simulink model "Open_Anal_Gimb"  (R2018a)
settings: Solver=ode5  StartTime=0.0  StopTime=25000  FixedStep=Ts  RelTol=1e-3  EnableMultiTasking=on
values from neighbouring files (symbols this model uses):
  Kq1 = I22*ww^2 - 3*wo2*(I11-I33)    [start.m]    (also in run.m)
  Kq2 = 2*I22*zet*ww    [start.m]    (also in run.m)
  Kqi = 0.0005    [start.m]    (also in run.m)
  Kr1 = (0.1*I11*I33*zet^2/Hy0) - sqrt( ((0.01^zet^4*I11^2*I33^2)/Hy0^2)+(4*I11*I33*zet^2) )    [start.m]    (also in run.m)
  Kr2 = 0.05*Kr1    [start.m]    (also in run.m)
  Kr3 = 0.04*zet*(Kr2-Hy0) * sqrt(abs(Hy0/(I11*I33)))    [start.m]    (also in run.m)
  Ts = 0.01    [start.m]    (also in run.m = 0.001; runf.m = 0.0005)
undefined symbols (not defined in the file or in its folder): Avf, Bvf, Cvf, den, DiscIntNeverNeededParam, Dvf, num, RW_Steering
libraries: simulink x3

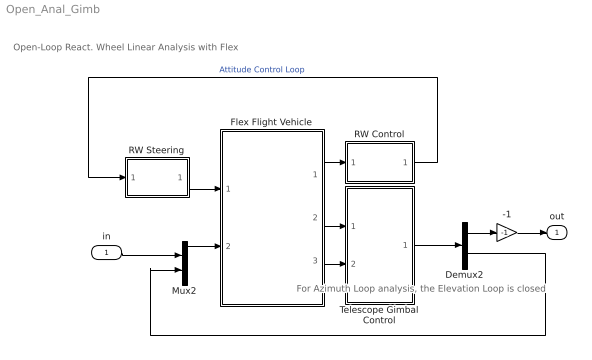
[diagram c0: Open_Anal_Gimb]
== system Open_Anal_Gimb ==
  note: For Azimuth Loop analysis, the Elevation Loop is closed
  note: Open-Loop React. Wheel Linear Analysis with Flex
  in : Inport
  -1 : Gain  Gain=-1
  Demux2 : Demux  Outputs=2
  Flex Flight Vehicle : Subsystem
  Mux2 : Mux  Inputs=2
  RW Control : Subsystem
  RW Steering : Subsystem
  Telescope Gimbal Control : Subsystem
  out : Outport
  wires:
  -1/1 -> out/1
  Flex Flight Vehicle/1(atti) -> RW Control/1(atti)
  RW Steering/1(Twi) -> Flex Flight Vehicle/1(Trw(i))
  Mux2/1 -> Flex Flight Vehicle/2(Tgimb)
  RW Control/1(Tc) -> RW Steering/1(Trwc)  "Attitude Control Loop"
  Flex Flight Vehicle/2(alfa) -> Telescope Gimbal Control/1(Gimb)
  Flex Flight Vehicle/3(alfad) -> Telescope Gimbal Control/2(Grate)
  Telescope Gimbal Control/1(GTrq) -> Demux2/1
  in/1 -> Mux2/1
  Demux2/1 -> -1/1
  Demux2/2 -> Mux2/2

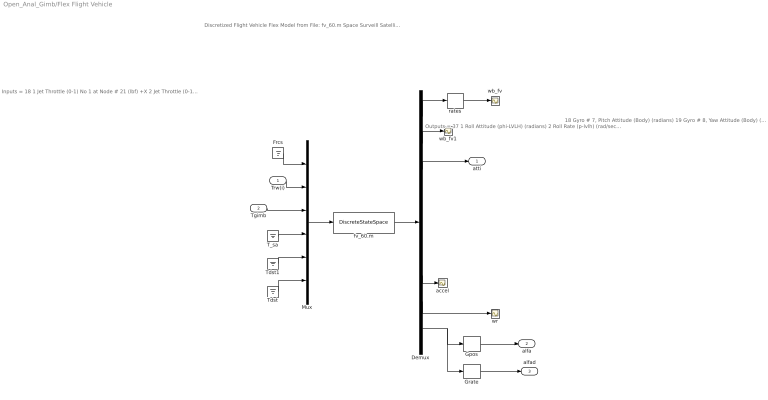
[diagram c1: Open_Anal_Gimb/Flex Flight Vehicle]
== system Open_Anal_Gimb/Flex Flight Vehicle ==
  note: Discretized Flight Vehicle Flex Model from File: fv_60.m Space Surveill Satellite with RCS and Reaction Wheels (Gimbals, 60 Modes, Z-Transf)
  note: Inputs = 18 1 Jet Throttle (0-1) No 1 at Node # 21 (lbf) +X 2 Jet Throttle (0-1) No 2 at Node # 22 (lbf) +X 3 Jet Throttle (0-1) No 3 at Node # 23 (lbf) +Y 4 Jet Throttle (0-1) No 4 at Node # 24 (lbf) -Y 5 Jet Throttle (0-1) No 5 at Node # 25 (lbf) -Y 6 Jet Throttle (0-1) No 6 at Node # 26 (lbf) +Y 7 Jet Throttle (0-1) No 7 at Node # 27 (lbf) +X 8 React-Wheel No 1 Torque to Spacecraft (ft-lb) 9 React-Wheel No 2 Torque to Spacecraft (ft-lb) 10 React-Wheel No 3 Torque to Spacecraft (ft-lb) 11 Elevation Trqu at Gimbal No 1 (ft-lb) 12 Azimuth Torque at Gimbal No 2 (ft-lb) 13 Rght SA Torque at Gimbal No 3 (ft-lb) 14 Left SA Torque at Gimbal No 4 (ft-lb) 15 Ext Torque Input 1 (ft-lb), dir: 1.00 0.00 0.00 16 Ext Torque Input 2 (ft-lb), dir: 0.00 1.00 0.00 17 Ext Torque Input 3 (ft-lb), dir: 0.00 0.00 1.00 18 Ext Torque Direct.=( 0.1970 -0.5964 -0.7782)
  note: Outputs = 37 1 Roll Attitude (phi-LVLH) (radians) 2 Roll Rate (p-lvlh) (rad/sec) 3 Pitch Attitude (thet-LVLH) (radians) 4 Pitch Rate (q-lvlh) (rad/sec) 5 Yaw Attitude (psi-LVLH) (radians) 6 Yaw Rate (r-lvlh) (rad/sec) 7 Angle of attack, alfa, (radians) 8 Angle of sideslip, beta, (radian) 9 Change in Altitude, delta-h, (feet) 10 Forward Acceleration (V-dot) (ft/sec) 11 Cross Range Velocity (Vcr) (ft/sec) 12 Rate-Gyro # 1, Roll Rate (Body) (rad/sec) 13 Rate-Gyro # 2, Pitch Rate (Body) (rad/sec) 14 Rate-Gyro # 3, Yaw Rate (Body) (rad/sec) 15 Gyro # 4, Roll Attitude (Body) (radians) 16 Gyro # 5, Pitch Attitude (Body) (radians) 17 Gyro # 6, Yaw Attitude (Body) (radians)
  note: 18 Gyro # 7, Pitch Attitude (Body) (radians) 19 Gyro # 8, Yaw Attitude (Body) (radians) 20 Gyro # 9, Pitch Attitude (Body) (radians) 21 Gyro # 10, Yaw Attitude (Body) (radians) 22 Gyro # 11, Roll Attitude (Body) (radians) 23 Gyro # 12, Pitch Attitude (Body) (radians) 24 Gyro # 13, Yaw Attitude (Body) (radians) 25 Translat. Accelerom # 1, (along X), (ft/sec^2) 26 Translat. Accelerom # 2, (along Y), (ft/sec^2) 27 Reaction Wheel # 1 Rate (rpm) relative to vehicle 28 Reaction Wheel # 2 Rate (rpm) relative to vehicle 29 Reaction Wheel # 3 Rate (rpm) relative to vehicle 30 Rotation Angle at Elevati Gimbal No 1 31 Rotation Rate at Elevati Gimbal No 1 32 Rotation Angle at Azimuth Gimbal No 2 33 Rotation Rate at Azimuth Gimbal No 2 34 Rotation Angle at Rght SA Gimbal No 3 35 Rotation Rate at Rght SA Gimbal No 3 36 Rotation Angle at Left SA Gimbal No 4 37 Rotation Rate at Left SA Gimbal No 4
  Trw(i) : Inport
  Tgimb : Inport  Port=2
  Demux : Demux  Outputs=[11, 3, 3, 2, 2, 3, 2, 3, 8]
  Frcs : Ground
  Gpos : Selector  InputPortWidth=8  IndexOptions=Index vector (dialog)  Indices=[1,3]  OutputSizes=1
  Grate : Selector  InputPortWidth=8  IndexOptions=Index vector (dialog)  Indices=[2,4]  OutputSizes=1
  Mux : Mux  Inputs=[7,3,2,2,3,1]
  T_sa : Ground
  Tdst : Ground
  Tdst1 : Ground
  accel : Scope
  fv_60.m : DiscreteStateSpace  A=Avf  B=Bvf  C=Cvf  D=Dvf  SampleTime=Ts
  rates : Selector  InputPortWidth=11  IndexOptions=Index vector (dialog)  Indices=[2, 4, 6]  OutputSizes=1
  wb_fv : Scope
  wb_fv1 : Scope
  wr : Scope
  atti : Outport
  alfa : Outport  Port=2
  alfad : Outport  Port=3
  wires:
  Mux/1 -> fv_60.m/1
  Frcs/1 -> Mux/1
  Trw(i)/1 -> Mux/2
  Demux/8 -> wr/1
  Demux/1 -> rates/1
  rates/1 -> wb_fv/1
  Demux/9 -> Gpos/1, Grate/1
  Demux/2 -> wb_fv1/1
  Demux/7 -> accel/1
  Demux/3 -> atti/1
  Grate/1 -> alfad/1
  Gpos/1 -> alfa/1
  Tgimb/1 -> Mux/3
  Tdst1/1 -> Mux/5
  T_sa/1 -> Mux/4
  Tdst/1 -> Mux/6
  fv_60.m/1 -> Demux/1

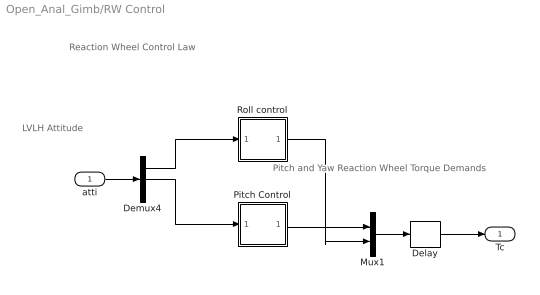
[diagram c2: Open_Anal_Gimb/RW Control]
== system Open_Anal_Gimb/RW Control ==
  note: Reaction Wheel Control Law
  note: LVLH Attitude
  note: Pitch and Yaw Reaction Wheel Torque Demands
  atti : Inport
  Delay : Delay  DelayLength=1  InputProcessing=Inherited  SampleTime=Ts
  Demux4 : Demux  Outputs=3
  Mux1 : Mux  Inputs=2
  Pitch Control : Subsystem
  Roll control : Subsystem
  Tc : Outport
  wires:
  Delay/1 -> Tc/1
  Roll control/1(Tcz) -> Mux1/2
  Mux1/1 -> Delay/1
  atti/1 -> Demux4/1
  Demux4/2 -> Pitch Control/1(the)
  Pitch Control/1(Tcy) -> Mux1/1
  Demux4/1 -> Roll control/1(phi)

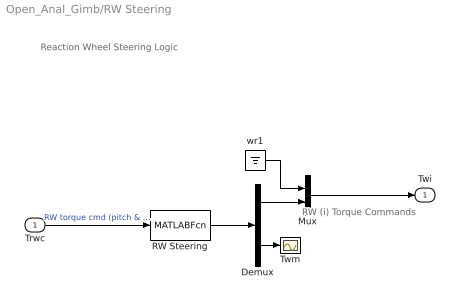
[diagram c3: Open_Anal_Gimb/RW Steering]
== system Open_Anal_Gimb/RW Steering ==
  note: Reaction Wheel Steering Logic
  note: RW (i) Torque Commands
  Trwc : Inport
  Demux : Demux  Outputs=[2, 1]
  Mux : Mux  Inputs=[1,2]
  RW Steering : MATLABFcn  MATLABFcn=RW_Steering( u(1:2) )  OutputDimensions=3
  Twm : Scope
  wr1 : Ground
  Twi : Outport
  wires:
  wr1/1 -> Mux/1
  Mux/1 -> Twi/1
  Trwc/1 -> RW Steering/1  "RW torque cmd (pitch & yaw)"
  RW Steering/1 -> Demux/1
  Demux/1 -> Mux/2
  Demux/2 -> Twm/1

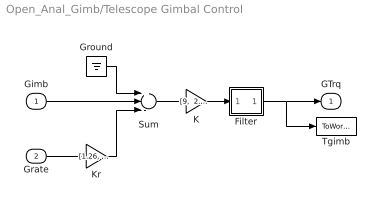
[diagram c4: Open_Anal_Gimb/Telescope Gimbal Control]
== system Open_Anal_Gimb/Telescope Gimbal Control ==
  Gimb : Inport
  Grate : Inport  Port=2
  Filter : Subsystem
  Ground : Ground
  K : Gain  Gain="[9,  2.85]"
  Kr : Gain  Gain="[1.26,  1.14]"
  Sum : Sum  Inputs=+--
  Tgimb : ToWorkspace  VariableName=Tgimb  SampleTime=-1
  GTrq : Outport
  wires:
  Sum/1 -> K/1
  Gimb/1 -> Sum/2
  Grate/1 -> Kr/1
  K/1 -> Filter/1(I)
  Kr/1 -> Sum/3
  Ground/1 -> Sum/1
  Filter/1(O) -> GTrq/1, Tgimb/1

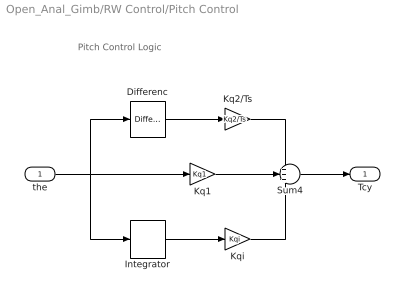
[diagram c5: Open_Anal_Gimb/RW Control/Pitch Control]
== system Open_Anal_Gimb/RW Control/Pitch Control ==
  note: Pitch Control Logic
  the : Inport
  Differenc : simulink/Discrete/Difference  ICPrevInput=0.0  InputProcessing=Inherited  OutMin=[]  OutMax=[]  OutDataType=sfix(16)  OutScaling=2^-10  DoSatur=off
  Integrator : DiscreteIntegrator  SampleTime=Ts  ICPrevOutput=DiscIntNeverNeededParam  ICPrevScaledInput=DiscIntNeverNeededParam
  Kq1 : Gain  Gain=Kq1
  Kq2/Ts : Gain  Gain=Kq2/Ts
  Kqi : Gain  Gain=Kqi
  Sum4 : Sum  Inputs=+++
  Tcy : Outport
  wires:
  Differenc/1 -> Kq2/Ts/1
  Integrator/1 -> Kqi/1
  Kqi/1 -> Sum4/3
  the/1 -> Differenc/1, Integrator/1, Kq1/1
  Kq2/Ts/1 -> Sum4/1
  Sum4/1 -> Tcy/1
  Kq1/1 -> Sum4/2

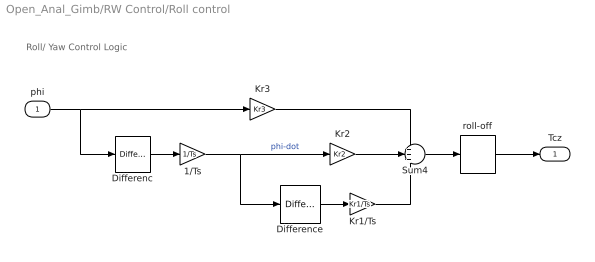
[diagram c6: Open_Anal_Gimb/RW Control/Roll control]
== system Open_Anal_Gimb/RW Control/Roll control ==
  note: Roll/ Yaw Control Logic
  phi : Inport
  1/Ts : Gain  Gain=1/Ts
  Differenc : simulink/Discrete/Difference  ICPrevInput=0.0  InputProcessing=Inherited  OutMin=[]  OutMax=[]  OutDataType=sfix(16)  OutScaling=2^-10  DoSatur=off
  Difference : simulink/Discrete/Difference  ICPrevInput=0.0  InputProcessing=Inherited  OutMin=[]  OutMax=[]  OutDataType=sfix(16)  OutScaling=2^-10  DoSatur=off
  Kr1/Ts : Gain  Gain=Kr1/Ts
  Kr2 : Gain  Gain=Kr2
  Kr3 : Gain  Gain=Kr3
  Sum4 : Sum  Inputs=+++
  roll-off : DiscreteTransferFcn  Numerator=[num]  Denominator=[den]  SampleTime=Ts
  Tcz : Outport
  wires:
  1/Ts/1 -> Difference/1, Kr2/1  "phi-dot"
  Differenc/1 -> 1/Ts/1
  Difference/1 -> Kr1/Ts/1
  Sum4/1 -> roll-off/1
  phi/1 -> Differenc/1, Kr3/1
  Kr1/Ts/1 -> Sum4/3
  Kr2/1 -> Sum4/2
  Kr3/1 -> Sum4/1
  roll-off/1 -> Tcz/1

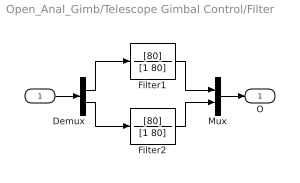
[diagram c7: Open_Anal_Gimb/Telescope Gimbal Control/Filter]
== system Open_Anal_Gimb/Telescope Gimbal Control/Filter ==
  I : Inport
  Demux : Demux  Outputs=2
  Filter1 : TransferFcn  Numerator=[80]  Denominator=[1 80]
  Filter2 : TransferFcn  Numerator=[80]  Denominator=[1 80]
  Mux : Mux  Inputs=2
  O : Outport
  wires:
  Mux/1 -> O/1
  I/1 -> Demux/1
  Demux/2 -> Filter2/1
  Demux/1 -> Filter1/1
  Filter2/1 -> Mux/2
  Filter1/1 -> Mux/1
